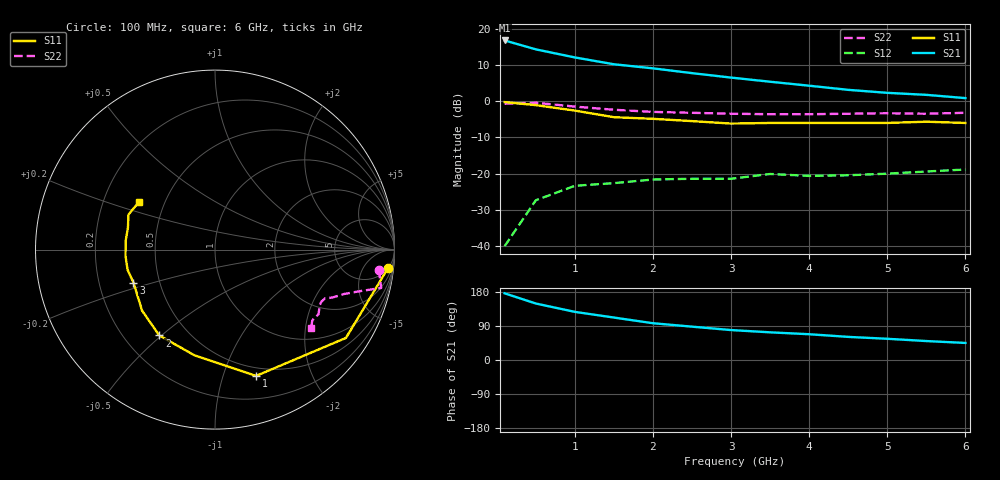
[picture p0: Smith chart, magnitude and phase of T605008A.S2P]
!AT-60500
!S-PARAMETERS at Vce=8V  Ic=2mA.  LAST UPDATED 07-21-92
!OBSOLETED Feb 1994 - nearest replacement: AT-41400
# ghz s ma r 50
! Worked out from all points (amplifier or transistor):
!   13 points, 100 MHz to 6 GHz, reference 50 ohm
!   highest |S21| = 16.7 dB at 100 MHz (marker M1)
!   |S21| within 3 dB of that: start of sweep to 621.9 MHz
!   unconditionally stable (mu >= 1): 2.901 GHz to end of sweep
!   at 1 GHz: K = 0.38, MSG = 17.7 dB, |S12| = -23.3 dB
!   at 3 GHz: K = 1.04, MAG = 12.7 dB, |S12| = -21.4 dB
!   at 6 GHz: K = 1.29, MAG = 6.6 dB, |S12| = -18.9 dB
!   lowest NFmin = 1.40 dB at 1 GHz
!   S11 on the Smith chart (normalised r, x): 100 MHz: 5, -18; 1 GHz: 0.41, -1.29; 2 GHz: 0.35, -0.49; 3 GHz: 0.35, -0.17; 6 GHz: 0.36, +0.25
0.1  0.97 -6.0  6.86 176.0  0.01 85.0  0.92 -7.0
0.5  0.88 -34.0  5.17 149.0  0.043 71.0  0.95 -13.0
1  0.74 -72.0  4 127.0  0.068 55.0  0.84 -16.0
1.5  0.6 -101.0  3.22 112.0  0.074 48.0  0.76 -19.0
2  0.57 -123.0  2.83 97.0  0.083 43.0  0.71 -22.0
2.5  0.53 -140.0  2.43 88.0  0.085 45.0  0.69 -23.0
3  0.49 -158.0  2.11 79.0  0.085 50.0  0.67 -24.0
3.5  0.5 -167.0  1.85 73.0  0.099 51.0  0.66 -26.0
4  0.5 -176.0  1.63 68.0  0.093 56.0  0.66 -28.0
4.5  0.5 174.0  1.43 61.0  0.095 58.0  0.67 -30.0
5  0.5 166.0  1.3 56.0  0.1 64.0  0.68 -32.0
5.5  0.52 158.0  1.22 50.0  0.107 67.0  0.67 -36.0
6  0.5 148.0  1.1 45.0  0.114 70.0  0.69 -39.0
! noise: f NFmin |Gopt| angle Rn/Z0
1  1.4  0.58  44  0.2
2  1.8  0.48  90  0.24
4  2.8  0.5  155  0.2
